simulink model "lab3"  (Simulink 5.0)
settings: Solver=ode5  StartTime=0.0  StopTime=50.0  FixedStep=0.01  RelTol=1e-3
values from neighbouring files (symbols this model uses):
  end_A = []    [Lab1_du.m]    (also in start.m = lab1_du(B_X, B_Y, 2))

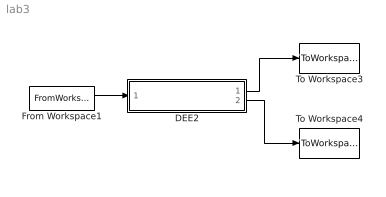
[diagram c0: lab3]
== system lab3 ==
  DEE2 : Subsystem
  From Workspace1 : FromWorkspace  VariableName=end_A  SampleTime=0
  To Workspace3 : ToWorkspace  VariableName=C_X  SampleTime=-1  SaveFormat=Array
  To Workspace4 : ToWorkspace  VariableName=C_Y  SampleTime=-1  SaveFormat=Array
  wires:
  DEE2/1(Port1) -> To Workspace3/1
  DEE2/2(Port2) -> To Workspace4/1
  From Workspace1/1 -> DEE2/1(SysInport1)

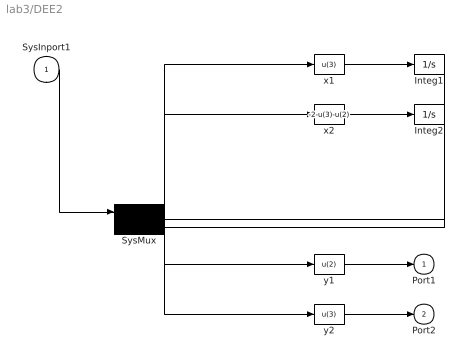
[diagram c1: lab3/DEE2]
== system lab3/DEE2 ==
  SysInport1 : Inport
  Integ1 : Integrator  InitialCondition=end_A(1)
  Integ2 : Integrator  InitialCondition=end_A(2)
  SysMux : Mux  Inputs=3
  x1 : Fcn  Expr=u(3)
  x2 : Fcn  Expr=-2-u(3)-u(2)
  y1 : Fcn  Expr=u(2)
  y2 : Fcn  Expr=u(3)
  Port1 : Outport
  Port2 : Outport  Port=2
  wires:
  SysInport1/1 -> SysMux/1
  SysMux/1 -> x1/1, x2/1, y1/1, y2/1
  x1/1 -> Integ1/1
  Integ1/1 -> SysMux/2
  x2/1 -> Integ2/1
  Integ2/1 -> SysMux/3
  y1/1 -> Port1/1
  y2/1 -> Port2/1
